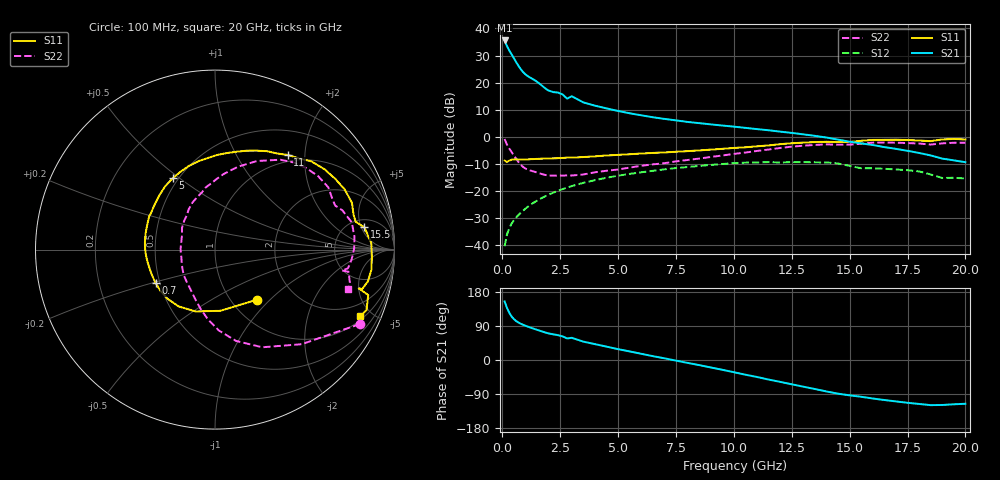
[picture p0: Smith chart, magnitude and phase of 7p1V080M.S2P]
! Infineon Technologies  Discrete & RF Semiconductors
! bfp620
! VCE =  1.0 V,  IC =  80 mA
! Common Emitter S-Parameters:  Sep 2002
# GHz  S  MA  R  50
!  f  S11  S21  S12  S22
! GHz  MAG  ANG  MAG  ANG  MAG  ANG  MAG  ANG
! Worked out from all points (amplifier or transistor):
!   59 points, 100 MHz to 20 GHz, reference 50 ohm
!   highest |S21| = 35.6 dB at 100 MHz (marker M1)
!   |S21| within 3 dB of that: start of sweep to 258.2 MHz
!   unconditionally stable (mu >= 1): 1.831 GHz to 2.377 GHz; 3.11 GHz to 10.56 GHz; 16.94 GHz to end of sweep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
!   at 1 GHz: K = 0.92, MSG = 24.8 dB, |S12| = -26.6 dB
!   at 5.5 GHz: K = 1.05, MAG = 9.9 dB, |S12| = -13.7 dB
!   at 20 GHz: K = 1.44, MAG = -0.9 dB, |S12| = -15.5 dB
!   S11 on the Smith chart (normalised r, x): 100 MHz: 1.30, -0.84; 700 MHz: 0.47, -0.21; 5 GHz: 0.47, +0.47; 11 GHz: 0.88, +1.67; 15.5 GHz: 6.69, +5.70; 20 GHz: 1.20, -4.28
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0.1  0.3632 -50.4  60.02 154.5  0.0095 74.4  0.9072 -27.2
0.2  0.3423 -85.0  47.34 138.0  0.0155 66.1  0.7149 -47.5
0.3  0.3614 -107.6  39.32 124.8  0.0204 63.4  0.6044 -64.2
0.4  0.3758 -122.6  33.24 115.0  0.0247 62.4  0.5223 -77.0
0.5  0.3809 -133.9  28.15 107.9  0.0285 62.0  0.4517 -87.2
0.6  0.381 -143.1  23.85 102.7  0.0322 61.9  0.3906 -95.8
0.7  0.3797 -150.7  20.34 98.8  0.0358 62.0  0.3407 -103.5
0.8  0.3788 -156.9  17.62 95.6  0.0394 62.0  0.3029 -110.5
1  0.38 -166.0  14.18 90.5  0.0469 61.9  0.2583 -122.4
1.4  0.3874 -177.6  11.05 81.6  0.0621 60.5  0.2249 -140.0
1.9  0.3953 169.4  7.579 71.8  0.081 57.1  0.195 -163.0
2.8  0.4112 153.0  5.043 56.9  0.1149 49.2  0.1924 168.8
3  0.4105 150.7  5.598 58.6  0.1224 47.3  0.1919 169.2
3.5  0.4211 142.4  4.301 48.5  0.1405 42.1  0.2003 156.6
5  0.4617 120.6  2.99 28.6  0.1906 26.5  0.2479 129.2
7  0.5118 94.4  2.134 4.5  0.2494 5.7  0.3243 103.5
10.5  0.6378 57.1  1.457 -38.8  0.3316 -34.8  0.51 69.4
11  0.6648 52.5  1.382 -44.8  0.3346 -40.5  0.5458 64.7
13.5  0.7969 24.8  1.037 -76.6  0.3369 -70.5  0.7053 35.5
15.5  0.8414 8.5  0.753 -97.0  0.2612 -92.4  0.7422 17.2
17  0.8787 -7.2  0.597 -109.3  0.2484 -101.5  0.7751 0.3
20  0.8903 -24.5  0.338 -115.5  0.1688 -112.1  0.7737 -16.3
